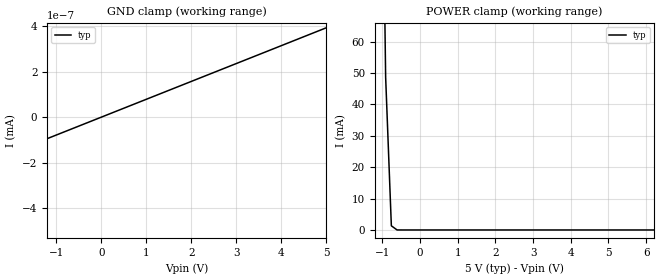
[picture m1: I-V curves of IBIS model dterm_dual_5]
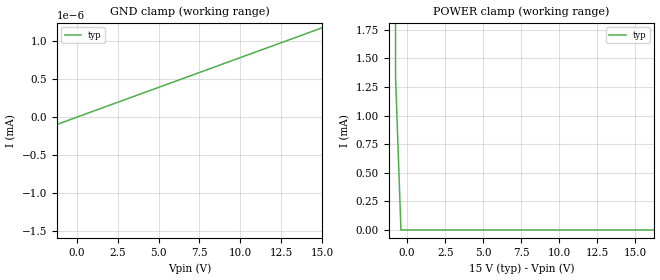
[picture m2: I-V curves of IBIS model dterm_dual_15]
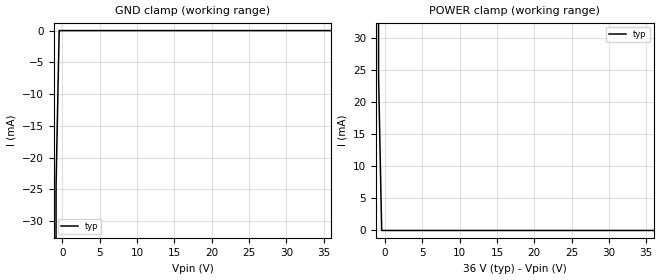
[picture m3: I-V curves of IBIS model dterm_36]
|Texas Instruments Incorporated
|tmux6201, 1 Data Lane 1:1 44V Precision mux
[IBIS Ver]   4.1
[File name]   tmux6201.ibs
[Date]   12/01/22
[File Rev]   1.0
[Source]
| Texas Instruments Incorporated.
| ASC-INT-MPD
| 12500 TI Blvd
| Dallas, TX - 75243
[Notes]   Revision History:
| Rev 1.0: 12/01/22
| - Initial version of the model
| - Model generated from simulations in SPECTRE
| - C_comp although listed in numerical order of value are
|   obtained from varying PVT conditions. For PVT conditions for
|   each specific value refer the buffer description under
|   respective [Model]. IBIS model user is responsible for using
|   appropriate C_comp to simulate for Signal Integrity.
[Disclaimer]
| This model is designed as an aid for customers of Texas Instruments.
| TI and its licensors and suppliers make no warranties, either expressed
| or implied, with respect to this  model, including the warranties of
| merchantability or fitness for a particular purpose. The model is
| provided solely on an "as is" basis. The entire risk as to its quality
| and performance is with the customer.
| This model is subject to change without notice. Texas Instruments
| Incorporated is not responsible for updating this model.
[Copyright]
(C) Copyright 2022 Texas Instruments Incorporated.All rights reserved.
|  Component TMUX6201DGK 8-pin - DGK package
|  Part # TMUX6201DGK
[Component]   TMUX6201DGK
[Manufacturer]  TI
[Package]
|   typ   min   max
R_pkg   0.0668   NA   NA
L_pkg   2.1992nH   NA   NA
C_pkg   0.2884pF   NA   NA
[Pin]   signal_name   model_name
   1   S   sterm
   2   NC   nc
   3   GND   gnd
   4   VDD   power
   5   NC   nc
   6   SEL   inbuf
   7   VSS   power
   8   D   dterm
[Series Switch Groups]
On 1 /
Off 1 /
[Series Pin Mapping]  pin_2 model_name function_table_group
   1   8   switch_dual_5   1
|   1   8   switch_dual_15   1
|   1   8   switch_36   1
|   1   8   switch_12   1
|  Component TMUX6201RQX 8-pin - RQX package
|  Part # TMUX6201RQX
[Component]   TMUX6201RQX
[Manufacturer]  TI
[Package]
|   typ   min   max
R_pkg   0.0668   NA   NA
L_pkg   2.1992nH   NA   NA
C_pkg   0.2884pF   NA   NA
[Pin]   signal_name   model_name
   1   S   sterm
   2   NC   nc
   3   GND   gnd
   4   VDD   power
   5   NC   nc
   6   SEL   inbuf
   7   VSS   power
   8   D   dterm
[Series Switch Groups]
On 1 /
Off 1 /
[Series Pin Mapping]  pin_2 model_name function_table_group
   1   8   switch_dual_5   1
|   1   8   switch_dual_15   1
|   1   8   switch_36   1
|   1   8   switch_12   1
[Model Selector] dterm
dterm_dual_5 Use for operation at +/-5V
dterm_dual_15 Use for operation at +/-15V
dterm_36 Use for operation at 36V
dterm_12 Use for operation at 12V
[Model Selector] sterm
sterm_dual_5 Use for operation at +/-5V
sterm_dual_15 Use for operation at +/-15V
sterm_36 Use for operation at 36V
sterm_12 Use for operation at 12V
[Model Selector] inbuf
inbuf_dual_5 Use for operation at +/-5V
inbuf_dual_15 Use for operation at +/-15V
inbuf_36 Use for operation at 36V
inbuf_12 Use for operation at 12V
| switch_dual_5
[Model]   switch_dual_5
Model_type   Series_switch
|   typ   min   max
C_comp   2.533030e-11   NA   NA
[Voltage Range]   5   NA   NA
[Power Clamp Reference]   5   NA   NA
[Temperature Range]   27   NA   NA
[On]
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[Off]
|   typ   min   max
[R Series]   10G   NA   NA
| switch_dual_15
[Model]   switch_dual_15
Model_type   Series_switch
|   typ   min   max
C_comp   4.014581e-11   NA   NA
[Voltage Range]   15   NA   NA
[Power Clamp Reference]   15   NA   NA
[Temperature Range]   27   NA   NA
[On]
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[Off]
|   typ   min   max
[R Series]   10G   NA   NA
| switch_36
[Model]   switch_36
Model_type   Series_switch
|   typ   min   max
C_comp   4.014581e-11   NA   NA
[Voltage Range]   36   NA   NA
[Power Clamp Reference]   36   NA   NA
[Temperature Range]   27   NA   NA
[On]
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[Off]
|   typ   min   max
[R Series]   10G   NA   NA
| switch_12
[Model]   switch_12
Model_type   Series_switch
|   typ   min   max
C_comp   2.533030e-11   NA   NA
[Voltage Range]   12   NA   NA
[Power Clamp Reference]   12   NA   NA
[Temperature Range]   27   NA   NA
[On]
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[Off]
|   typ   min   max
[R Series]   10G   NA   NA
| Models and submodels in the file (16): dterm_dual_5 (Terminator), dterm_dual_15 (Terminator), dterm_36 (Terminator), dterm_12 (Terminator), switch_dual_5 (Series_switch), switch_dual_15 (Series_switch), switch_36 (Series_switch), switch_12 (Series_switch), sterm_dual_5 (Terminator), sterm_dual_15 (Terminator), sterm_36 (Terminator), sterm_12 (Terminator), inbuf_dual_5 (Input), inbuf_dual_15 (Input), inbuf_36 (Input), inbuf_12 (Input)
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| dterm_dual_5
[Model]   dterm_dual_5
Model_type   Terminator
|   typ   min   max
C_comp   2.533030e-11   NA   NA
[Voltage Range]   5   NA   NA
[Temperature Range]   27   NA   NA
[Power Clamp Reference]   5   NA   NA
[GND Clamp Reference]   0   NA   NA
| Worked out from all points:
|   GND clamp passes 1 mA (typ) near -5.72 V on its own axis
|   POWER clamp passes 1 mA (typ) near -0.72 V on its own axis
[GND Clamp]
|   Voltage   I(typ)   I(min)   I(max)
-10V      -11.28A    NA         NA
-5.303V   -789.4pA   NA         NA
-5.152V   -411pA     NA         NA
-5V       -394.1pA   NA         NA
5V        393.6pA    NA         NA
[POWER Clamp]
|   Voltage   I(typ)   I(min)   I(max)
-5V       13.24A     NA         NA
-1.061V   184.2mA    NA         NA
-909.1mV  48.72mA    NA         NA
-757.6mV  1.324mA    NA         NA
-606.1mV  6.572uA    NA         NA
10V       -394.1pA   NA         NA
| dterm_dual_15
[Model]   dterm_dual_15
Model_type   Terminator
|   typ   min   max
C_comp   4.014581e-11   NA   NA
[Voltage Range]   15   NA   NA
[Temperature Range]   27   NA   NA
[Power Clamp Reference]   15   NA   NA
[GND Clamp Reference]   0   NA   NA
[GND Clamp]
|   Voltage   I(typ)   I(min)   I(max)
-20V      -11.55A    NA         NA
-15.4V    -9.307nA   NA         NA
-15.05V   -1.181nA   NA         NA
15V       1.176nA    NA         NA
[POWER Clamp]
|   Voltage   I(typ)   I(min)   I(max)
-5V       13.26A     NA         NA
-1.111V   275.7mA    NA         NA
-757.6mV  1.337mA    NA         NA
-404mV    6.544nA    NA         NA
30V       -1.177nA   NA         NA
| dterm_36
[Model]   dterm_36
Model_type   Terminator
|   typ   min   max
C_comp   4.014581e-11   NA   NA
[Voltage Range]   36   NA   NA
[Temperature Range]   27   NA   NA
[Power Clamp Reference]   36   NA   NA
[GND Clamp Reference]   0   NA   NA
[GND Clamp]
|   Voltage   I(typ)   I(min)   I(max)
-5V       -11.6A     NA         NA
-1.273V   -621mA     NA         NA
-858.6mV  -24.19mA   NA         NA
-444.4mV  -30.96nA   NA         NA
36V       1.41nA     NA         NA
[POWER Clamp]
|   Voltage   I(typ)   I(min)   I(max)
-5V       13.26A     NA         NA
-1.273V   611.4mA    NA         NA
-858.6mV  23.93mA    NA         NA
-444.4mV  23.28nA    NA         NA
36V       -1.411nA   NA         NA
